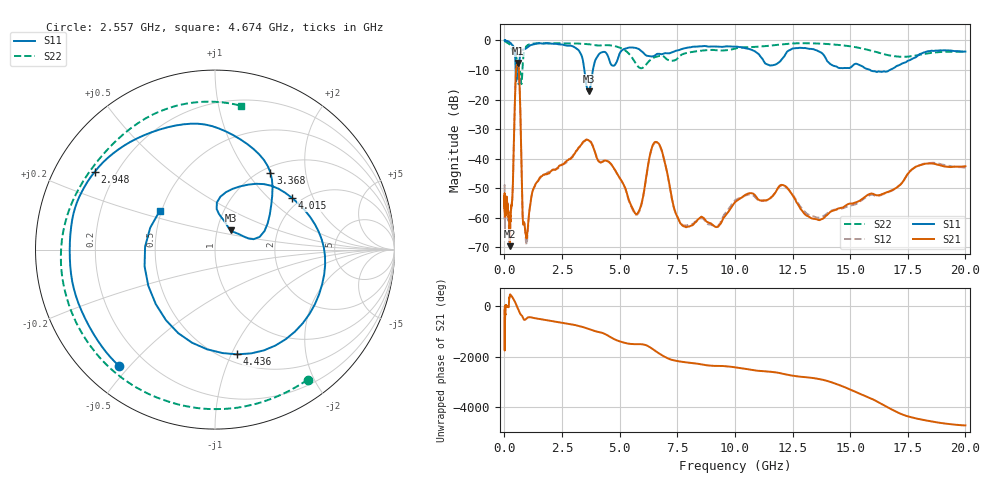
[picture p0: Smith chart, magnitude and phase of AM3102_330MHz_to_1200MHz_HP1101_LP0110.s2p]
! Date/Time: Tue, Sep 11, 2018 5:22 PM
! Network Analyzer: Agilent Technologies E8362B Rev: A.07.50.63
! Sweep from 0.010 to 20.000 GHz, 1601 Points, Sweep Type: LOG
! Power Supply: 4.949 V, 0.001 A
# Hz S DB R 50
!freq MagS11 AngS11 MagS21 AngS21 MagS12 AngS12 MagS22 AngS22
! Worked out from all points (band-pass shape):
!   1601 points, 10 MHz to 20 GHz, reference 50 ohm
!   highest |S21| = -7.63 dB at 580.7 MHz (marker M1); lowest = -69.6 dB at 240 MHz (marker M2)
!   |S21| within 3 dB of the highest: 502 MHz to 634.3 MHz (132.3 MHz wide, 23.3 % of centre)
!   lowest |S11| = -17.2 dB at 3.651 GHz (marker M3), VSWR 1.32, Z = 58.1 + j12.6 ohm
!   |S11| at or under -10 dB: 487 MHz to 547.1 MHz (60.02 MHz wide, 11.6 % of centre); 3.471 GHz to 3.841 GHz (370.7 MHz wide, 10.1 % of centre); 15.86 GHz to 16.73 GHz (870.2 MHz wide, 5.34 % of centre)
!   |S22| runs from -14.9 to -0.2 dB; largest |S21 - S12| = 0.0058
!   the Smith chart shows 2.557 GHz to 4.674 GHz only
!   S11 on the Smith chart (normalised r, x): 2.557 GHz: 0.11, -0.47; 2.948 GHz: 0.12, +0.29; 3.368 GHz: 1.09, +1.30; 4.015 GHz: 1.80, +1.41; 4.436 GHz: 0.58, -1.06; 4.674 GHz: 0.49, +0.25
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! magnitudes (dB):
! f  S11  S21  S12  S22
! 10 MHz  0.0  -52.7  -49.0  -0.2
! 35.55 MHz  -0.1  -58.6  -58.4  -0.3
! 126.4 MHz  -0.2  -56.2  -55.1  -0.8
! 240 MHz  -0.7  -69.6  -67.8  -1.4
! 356 MHz  -1.7  -51.4  -52.0  -3.8
! 447.2 MHz  -3.6  -23.1  -23.1  -4.3
! 580.7 MHz  -9.1  -7.6  -7.7  -10.5
! 666.5 MHz  -5.4  -16.7  -16.7  -10.9
! 798.4 MHz  -3.2  -60.4  -60.4  -7.8
! 942.8 MHz  -2.7  -66.6  -68.4  -2.1
! 1.59 GHz  -1.1  -46.0  -46.1  -1.0
! 2.557 GHz  -1.5  -41.9  -41.9  -1.0
! 2.948 GHz  -2.0  -39.5  -39.2  -1.0
! 3.368 GHz  -5.5  -34.9  -35.0  -1.2
! 3.651 GHz  -17.2  -33.8  -33.5  -1.3
! 4.015 GHz  -5.7  -39.8  -39.6  -1.7
! 4.436 GHz  -4.5  -40.7  -40.6  -1.6
! 4.674 GHz  -8.5  -42.3  -42.4  -1.8
! 5.652 GHz  -2.5  -58.2  -58.4  -7.2
! 6.58 GHz  -4.8  -34.3  -34.5  -5.5
! 7.92 GHz  -2.5  -63.1  -62.5  -4.2
! 20 GHz  -3.8  -42.6  -43.0  -3.9
